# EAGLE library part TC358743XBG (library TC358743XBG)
Display Drivers & Controllers HDMI to CSI-2 bridge chip Source: Datasheet
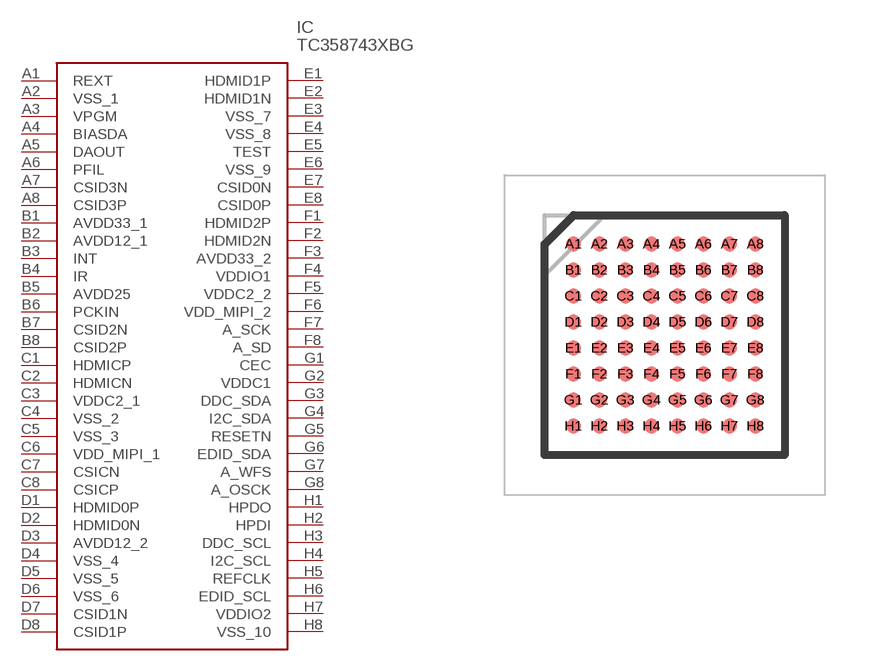
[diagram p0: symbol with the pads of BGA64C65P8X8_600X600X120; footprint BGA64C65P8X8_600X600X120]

Designator prefix IC

## TC358743XBG (Description: Display Drivers & Controllers HDMI to CSI-2 bridge chip; Height: 1.2mm; Manufacturer_Name: Toshiba; Manufacturer_Part_Number: TC358743XBG)  [BGA64C65P8X8_600X600X120]
A1  REXT
A2  VSS_1
A3  VPGM
A4  BIASDA
A5  DAOUT
A6  PFIL
A7  CSID3N
A8  CSID3P
B1  AVDD33_1
B2  AVDD12_1
B3  INT
B4  IR
B5  AVDD25
B6  PCKIN
B7  CSID2N
B8  CSID2P
C1  HDMICP
C2  HDMICN
C3  VDDC2_1
C4  VSS_2
C5  VSS_3
C6  VDD_MIPI_1
C7  CSICN
C8  CSICP
D1  HDMID0P
D2  HDMID0N
D3  AVDD12_2
D4  VSS_4
D5  VSS_5
D6  VSS_6
D7  CSID1N
D8  CSID1P
E1  HDMID1P
E2  HDMID1N
E3  VSS_7
E4  VSS_8
E5  TEST
E6  VSS_9
E7  CSID0N
E8  CSID0P
F1  HDMID2P
F2  HDMID2N
F3  AVDD33_2
F4  VDDIO1
F5  VDDC2_2
F6  VDD_MIPI_2
F7  A_SCK
F8  A_SD
G1  CEC
G2  VDDC1
G3  DDC_SDA
G4  I2C_SDA
G5  RESETN
G6  EDID_SDA
G7  A_WFS
G8  A_OSCK
H1  HPDO
H2  HPDI
H3  DDC_SCL
H4  I2C_SCL
H5  REFCLK
H6  EDID_SCL
H7  VDDIO2
H8  VSS_10

## Footprint BGA64C65P8X8_600X600X120 (pad centres in mm)
P-TFBGA64-0606-0.65-001
smd 0.37 x 0.37: A1 -2.275,2.275; A2 -1.625,2.275; A3 -0.975,2.275; A4 -0.325,2.275; A5 0.325,2.275; A6 0.975,2.275; A7 1.625,2.275; A8 2.275,2.275; B1 -2.275,1.625; B2 -1.625,1.625; B3 -0.975,1.625; B4 -0.325,1.625; B5 0.325,1.625; B6 0.975,1.625; B7 1.625,1.625; B8 2.275,1.625; C1 -2.275,0.975; C2 -1.625,0.975; C3 -0.975,0.975; C4 -0.325,0.975; C5 0.325,0.975; C6 0.975,0.975; C7 1.625,0.975; C8 2.275,0.975; D1 -2.275,0.325; D2 -1.625,0.325; D3 -0.975,0.325; D4 -0.325,0.325; D5 0.325,0.325; D6 0.975,0.325; D7 1.625,0.325; D8 2.275,0.325; E1 -2.275,-0.325; E2 -1.625,-0.325; E3 -0.975,-0.325; E4 -0.325,-0.325; E5 0.325,-0.325; E6 0.975,-0.325; E7 1.625,-0.325; E8 2.275,-0.325; F1 -2.275,-0.975; F2 -1.625,-0.975; F3 -0.975,-0.975; F4 -0.325,-0.975; F5 0.325,-0.975; F6 0.975,-0.975; F7 1.625,-0.975; F8 2.275,-0.975; G1 -2.275,-1.625; G2 -1.625,-1.625; G3 -0.975,-1.625; G4 -0.325,-1.625; G5 0.325,-1.625; G6 0.975,-1.625; G7 1.625,-1.625; G8 2.275,-1.625; H1 -2.275,-2.275; H2 -1.625,-2.275; H3 -0.975,-2.275; H4 -0.325,-2.275; H5 0.325,-2.275; H6 0.975,-2.275; H7 1.625,-2.275; H8 2.275,-2.275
